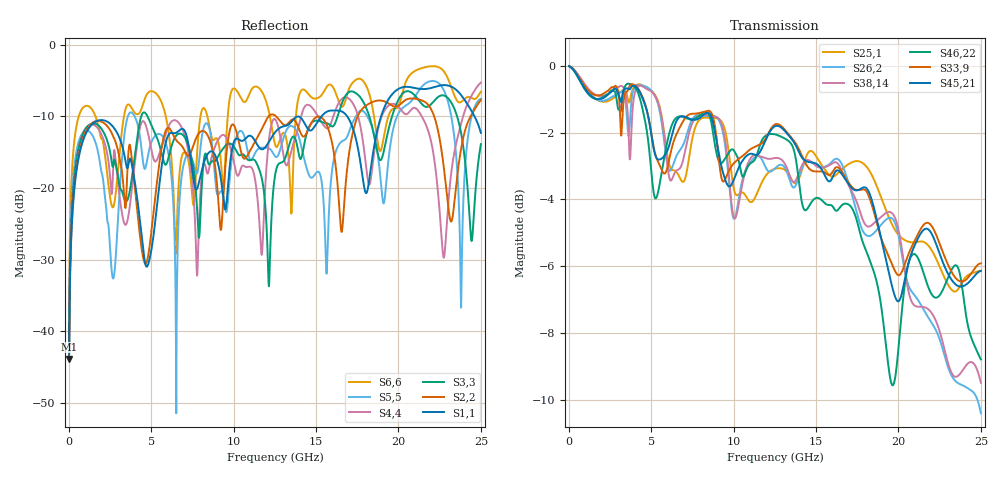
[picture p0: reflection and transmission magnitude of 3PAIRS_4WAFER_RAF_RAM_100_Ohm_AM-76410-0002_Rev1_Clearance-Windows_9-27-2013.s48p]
! Model Description:  Impact 3 pair RAF RAM 4 wafer 100 Ohm mated connector
! Molex Part Number: 76410-series (RAM), 76170-series
! (daughter card connector)
! IMPORTANT NOTE: This model should not be used to evaluate
! electrical signals with a greater than 25 GHz. of frequency content.
! Please apply appropriate analysis techniques when reviewing the results of
! your simulations.
!  COPYRIGHT 2008, BY MOLEX INCORPORATED
!  ALL INTERNATIONAL RIGHTS RESERVED
!  THIS FILE CONTAINS MOLEX INCORPORATED CONFIDENTIAL INFORMATION
! >>>>>>>>>>>>>>>>  USER AGREEMENT  <<<<<<<<<<<<<<<<<<<
! The information on this media is the property of MOLEX Incorporated
! and  has been provided to you free of charge. Molex does not
! guarantee that the information is error-free, nor does MOLEX  make
! any representations, warranty or guarantee that the information is
! accurate, correct, reliable or up-to-date. MOLEX expressly
! disclaims all implied warranties regarding this information,
! including but not limited to any implied  warranties of
! merchantability or fitness for a particular purpose. MOLEX does
! not warrant that the media will work correctly in your multi- user
! or network environment.
! MOLEX will in no case be liable for your use, or the results of
! your use, of the software and other information contained on this
! media or  any accompanying written materials.  IT IS YOUR
! RESPONSIBILITY TO VERIFY THE RESULTS OF YOUR USE OF THIS
! INFORMATION IN YOUR OWN PARTICULAR ENGINEERING AND PRODUCT
! ENVIRONMENT, AND YOU ASSUME THE ENTIRE RISK OF DOING SO OR
! FAILING TO DO SO.  In no event will MOLEX be liable for any
! direct, indirect, incidental or consequential damages arising from
! your use of, or your inability to use, software, product simulations
! and other information contained on this media or any accompanying
! written materials.
! This model has not been validated with empirical data.
! This model was solved using HFSS.  TDR results can run 5-8 ohms low
! Touchstone file from project 3PAIRS_4WAFER_RAF_RAM_100_Ohm_AM-76410-0002_Rev1_Clearance-Windows_9-27-2013
! Exported from HFSS 15.0.0
! Variables:
!  wplen = 1mm
! Terminal data exported
! Port[1] = B1_T1
! Port[2] = C1_T1
! Port[3] = E1_T1
! Port[4] = F1_T1
! Port[5] = H1_T1
! Port[6] = J1_T1
! Port[7] = A2_T1
! Port[8] = B2_T1
! Port[9] = D2_T1
! Port[10] = E2_T1
! Port[11] = G2_T1
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# GHZ S MA R 50.000000
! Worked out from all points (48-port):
!   1250 points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, 20 MHz to 25 GHz, reference 50 ohm
!   strongest paths, dB at 20 MHz, 6.26 GHz, 12.52 GHz, 18.76 GHz, 25 GHz:
!     S45,21: 0.0, -2.1, -1.8, -4.8, -6.1
!     S33,9: 0.0, -2.4, -1.8, -4.8, -5.9
!     S46,22: 0.0, -1.8, -2.1, -6.6, -8.8
!     S38,14: 0.0, -3.4, -2.8, -4.6, -9.5
!     S26,2: 0.0, -3.1, -3.1, -4.9, -10.4
!     S25,1: 0.0, -3.1, -3.1, -3.7, -6.1
!   lowest |S11| = -43.8 dB at 20 MHz (marker M1), VSWR 1.01, Z = 50 + j0.643 ohm
!   |S11| at or under -10 dB: start of sweep to 15.32 GHz; 16.89 GHz to 18.94 GHz (2.049 GHz wide, 11.4 % of centre); 24.62 GHz to end of sweep
